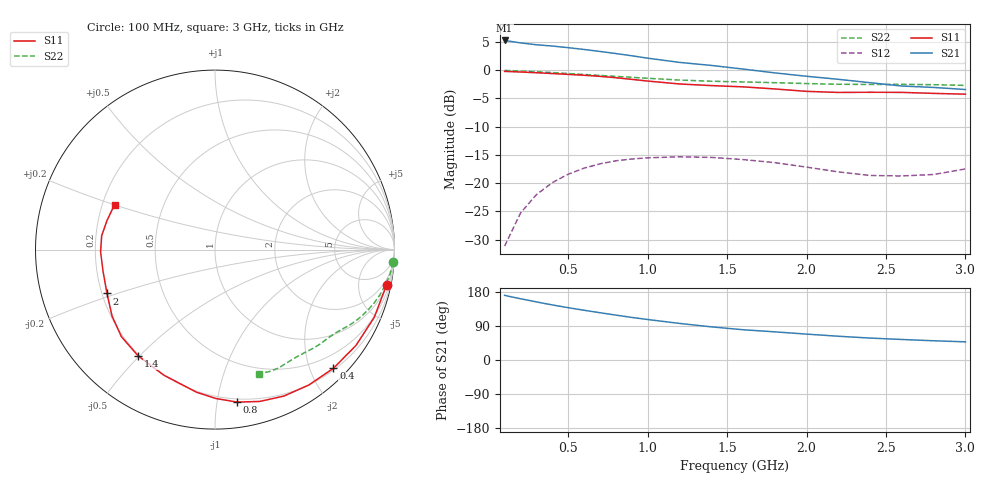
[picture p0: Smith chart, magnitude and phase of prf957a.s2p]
! Filename:  PRF957A.S2P  Version:  3.0
! Philips part #:  PRF957  Date:  Nov 1998
! Bias condition:  Vce=3V, Ic=0.5mA
#  MHz  S  MA  R 50
! Freq  S11  S21  S12  S22
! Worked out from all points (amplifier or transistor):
!   20 points, 100 MHz to 3 GHz, reference 50 ohm
!   highest |S21| = 5.3 dB at 100 MHz (marker M1)
!   |S21| within 3 dB of that: start of sweep to 967.7 MHz
!   unconditionally stable (mu >= 1): 2.287 GHz to end of sweep
!   at 400 MHz: K = 0.13, MSG = 12.1 dB, |S12| = -19.9 dB
!   at 1.2 GHz: K = 0.39, MSG = 8.4 dB, |S12| = -15.3 dB
!   at 3 GHz: K = 1.28, MAG = 3.9 dB, |S12| = -17.5 dB
!   S11 on the Smith chart (normalised r, x): 100 MHz: 1.16, -9.63; 400 MHz: 0.23, -2.39; 800 MHz: 0.18, -1.14; 1.4 GHz: 0.19, -0.50; 2 GHz: 0.22, -0.19; 3 GHz: 0.25, +0.20
100  0.9759 -11.7  1.834 170.5  0.02763 82.5  0.9954 -4.1
200  0.9642 -23.0  1.745 161.7  0.0543 76.0  0.9843 -8.0
300  0.9498 -34.2  1.68 153.3  0.079 69.7  0.9698 -11.8
400  0.9342 -45.0  1.637 145.4  0.1009 63.7  0.953 -15.3
500  0.918 -55.3  1.584 138.0  0.1199 58.5  0.9349 -18.6
600  0.9018 -64.8  1.526 131.2  0.1356 53.7  0.9163 -21.5
700  0.882 -73.6  1.466 124.8  0.1482 49.3  0.8991 -24.1
800  0.8582 -81.8  1.405 118.5  0.1576 45.2  0.8819 -26.4
900  0.8295 -89.7  1.342 112.3  0.1634 41.5  0.8651 -28.6
1000  0.8016 -97.3  1.278 106.9  0.1675 38.3  0.8482 -30.6
1200  0.7552 -112.2  1.173 96.6  0.1709 32.7  0.8181 -34.4
1400  0.7307 -125.9  1.102 87.5  0.1689 28.2  0.7986 -38.3
1600  0.7121 -137.1  1.024 79.9  0.1616 26.1  0.7871 -42.0
1800  0.6825 -147.2  0.9469 74.3  0.1519 26.1  0.7753 -45.3
2000  0.6495 -157.9  0.8837 68.3  0.1386 27.5  0.7615 -48.8
2200  0.6353 -169.1  0.8304 62.7  0.1257 31.5  0.7505 -53.0
2400  0.6375 -178.9  0.7753 57.9  0.1169 38.9  0.7472 -57.6
2600  0.6361 173.0  0.7241 54.2  0.1157 49.7  0.7489 -61.9
2800  0.6231 165.0  0.7035 50.8  0.1192 61.8  0.7442 -66.0
3000  0.6133 155.9  0.6745 47.9  0.1335 72.7  0.7334 -70.5
